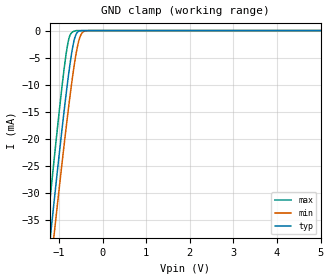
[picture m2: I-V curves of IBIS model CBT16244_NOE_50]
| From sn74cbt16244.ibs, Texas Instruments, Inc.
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[Model]   CBT16244_NOE_50
Model_type  Input
Vinl = 0.8
Vinh = 2.0
| variable   typ   min   max
C_comp   1.66pF   1.08pF   4.74pF
[Temperature Range]   40   100   -40
| Ambient temperature   25   85   -40
[Voltage range]   5   4.5   5.5
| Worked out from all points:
|   GND clamp passes 1 mA (typ) near -0.62 V on its own axis
[GND Clamp]
| CBT16244_NOE_50
|   Voltage   I(typ)   I(min)   I(max)
-5V       -348.8mA   -347.8mA   -351.9mA
-1.31V    -46.71mA   -52.51mA   -39.5mA
-1.27V    -43.61mA   -49.48mA   -36.29mA
-1.195V   -37.84mA   -43.83mA   -30.32mA
-1.095V   -30.24mA   -36.39mA   -22.5mA
-925mV    -17.78mA   -24.08mA   -9.91mA
-820mV    -10.62mA   -16.82mA   -3.428mA
-755mV    -6.612mA   -12.56mA   -1.035mA
-660mV    -2.039mA   -6.894mA   -131.8uA
-525mV    -67.19uA   -1.329mA   -198.8nA
-380mV    -784.8nA   -49.31uA   -584.8pA
5V        40.84pA    2.728nA    29.22pA
